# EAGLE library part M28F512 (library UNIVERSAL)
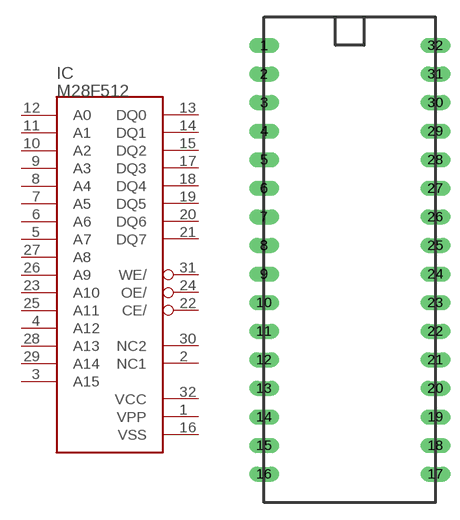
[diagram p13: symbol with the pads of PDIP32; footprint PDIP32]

Designator prefix IC

## M28F512  [PDIP32]
1  VPP  pwr
2  NC1  nc
3  A15  in
4  A12  in
5  A7  in
6  A6  in
7  A5  in
8  A4  in
9  A3  in
10  A2  in
11  A1  in
12  A0  in
13  DQ0
14  DQ1
15  DQ2
16  VSS  sup
17  DQ3
18  DQ4
19  DQ5
20  DQ6
21  DQ7
22  CE/  in
23  A10
24  OE/  in
25  A11
26  A9
27  A8
28  A13
29  A14
30  NC2  nc
31  WE/  in
32  VCC  sup

## Footprint PDIP32 (pad centres in mm)
drill 0.813 pad 1.092 long: 1 0,2.54; 2 0,0; 3 0,-2.54; 4 0,-5.08; 5 0,-7.62; 6 0,-10.16; 7 0,-12.7; 8 0,-15.24; 9 0,-17.78; 10 0,-20.32; 11 0,-22.86; 12 0,-25.4; 13 0,-27.94; 14 0,-30.48; 15 0,-33.02; 16 0,-35.56; 17 15.24,-35.56; 18 15.24,-33.02; 19 15.24,-30.48; 20 15.24,-27.94; 21 15.24,-25.4; 22 15.24,-22.86; 23 15.24,-20.32; 24 15.24,-17.78; 25 15.24,-15.24; 26 15.24,-12.7; 27 15.24,-10.16; 28 15.24,-7.62; 29 15.24,-5.08; 30 15.24,-2.54; 31 15.24,0; 32 15.24,2.54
